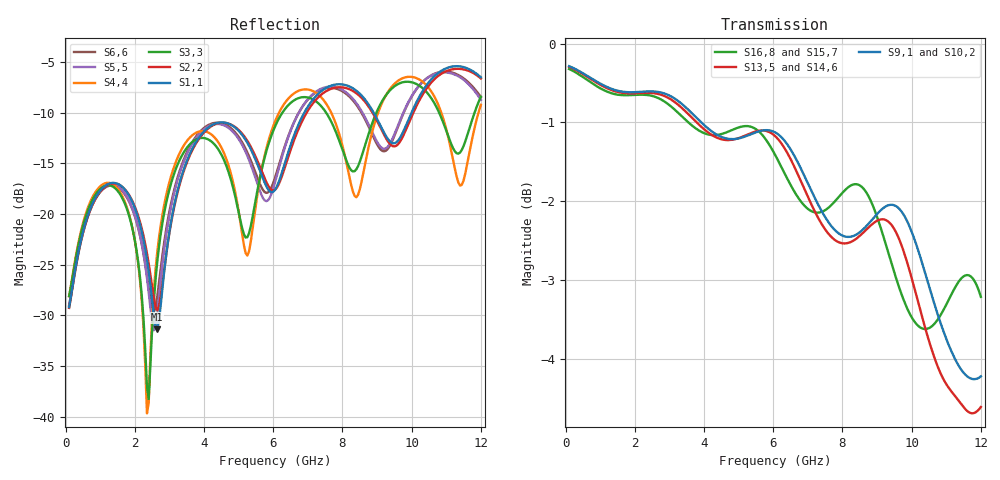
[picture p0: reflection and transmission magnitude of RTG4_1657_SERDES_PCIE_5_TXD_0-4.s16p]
! RTG4 1657 S-parameter file
! Microsemi Corporation (c) 2019
!Initial ver: Jul 30, 2019
! Port::PIN_NAME::NET_NAME::S-parameter ports::PORT SIDE
! Port1:--:SERDES_PCIE_5_TXD0_N_DIE::1::DIE
! Port2:--:SERDES_PCIE_5_TXD0_P_DIE::2::DIE
! Port3:AW34:SERDES_PCIE_5_TXD0_N_BGA::3::BGA
! Port4:AV34:SERDES_PCIE_5_TXD0_P_BGA::4::BGA
! Port5:--:SERDES_PCIE_5_TXD1_N_DIE::5::DIE
! Port6:--:SERDES_PCIE_5_TXD1_P_DIE::6::DIE
! Port7:AW36:SERDES_PCIE_5_TXD1_N_BGA::7::BGA
! Port8:AV36:SERDES_PCIE_5_TXD1_P_BGA::8::BGA
! Port9:--:SERDES_PCIE_5_TXD2_N_DIE::9::DIE
! Port10:--:SERDES_PCIE_5_TXD2_P_DIE::10::DIE
! Port11:AU37:SERDES_PCIE_5_TXD2_N_BGA::11::BGA
! Port12:AT37:SERDES_PCIE_5_TXD2_P_BGA::12::BGA
! Port13:--:SERDES_PCIE_5_TXD3_N_DIE::13::DIE
! Port14:--:SERDES_PCIE_5_TXD3_P_DIE::14::DIE
! Port15:AU39:SERDES_PCIE_5_TXD3_N_BGA::15::BGA
! Port16:AT39:SERDES_PCIE_5_TXD3_P_BGA::16::BGA
!TouchstoneFormatFlag = 1
! GNDNET
! NETSLIST
! User Comments:
! Touchstone file exported from HFSS 2018.2.0
!  File:  //LSI_Z840_SIM_PC/Simulation_Data/MASUMISU/Microsemi_190710/YBD197_150320_NETCHANGE_SERDES_PCIE_5_TXD.aedt
!  Generated:  12:49:29 ??  7 18, 2019
!  Design:  HFSSModel1
!  Project:  YBD197_150320_NETCHANGE_SERDES_PCIE_5_TXD
!  Setup:  Setup1
!  Solution:  Sweep
! Terminal data exported
! Port[1] = SERDES_PCIE_5_TXD0_N_DIE
! Port[2] = SERDES_PCIE_5_TXD0_P_DIE
! Port[3] = SERDES_PCIE_5_TXD1_N_DIE
! Port[4] = SERDES_PCIE_5_TXD1_P_DIE
! Port[5] = SERDES_PCIE_5_TXD2_N_DIE
! Port[6] = SERDES_PCIE_5_TXD2_P_DIE
! Port[7] = SERDES_PCIE_5_TXD3_N_DIE
! Port[8] = SERDES_PCIE_5_TXD3_P_DIE
! Port[9] = SERDES_PCIE_5_TXD0_N_BGA
! Port[10] = SERDES_PCIE_5_TXD0_P_BGA
! Port[11] = SERDES_PCIE_5_TXD1_N_BGA
! Port[12] = SERDES_PCIE_5_TXD1_P_BGA
! Port[13] = SERDES_PCIE_5_TXD2_N_BGA
! Port[14] = SERDES_PCIE_5_TXD2_P_BGA
! Port[15] = SERDES_PCIE_5_TXD3_N_BGA
! Port[16] = SERDES_PCIE_5_TXD3_P_BGA
# GHZ S DB R 50.000000
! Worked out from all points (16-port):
!   239 points, 100 MHz to 12 GHz, reference 50 ohm
!   strongest paths, dB at 100 MHz, 3.05 GHz, 6.05 GHz, 9.05 GHz, 12 GHz:
!     S9,1: -0.3, -0.7, -1.1, -2.1, -4.2
!     S13,5: -0.3, -0.7, -1.2, -2.2, -4.6
!     S10,2: -0.3, -0.7, -1.2, -2.2, -4.2
!     S14,6: -0.3, -0.7, -1.3, -2.4, -4.5
!     S16,8: -0.3, -0.8, -1.4, -2.3, -3.2
!     S15,7: -0.3, -0.8, -1.5, -2.5, -3.5
!   lowest |S11| = -31.4 dB at 2.65 GHz (marker M1), VSWR 1.06, Z = 52.3 + j1.56 ohm
!   |S11| at or under -10 dB: start of sweep to 6.894 GHz; 8.902 GHz to 9.996 GHz (1.093 GHz wide, 11.6 % of centre)
